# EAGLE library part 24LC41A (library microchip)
Serial EEPROM 128/512 byte, dual port
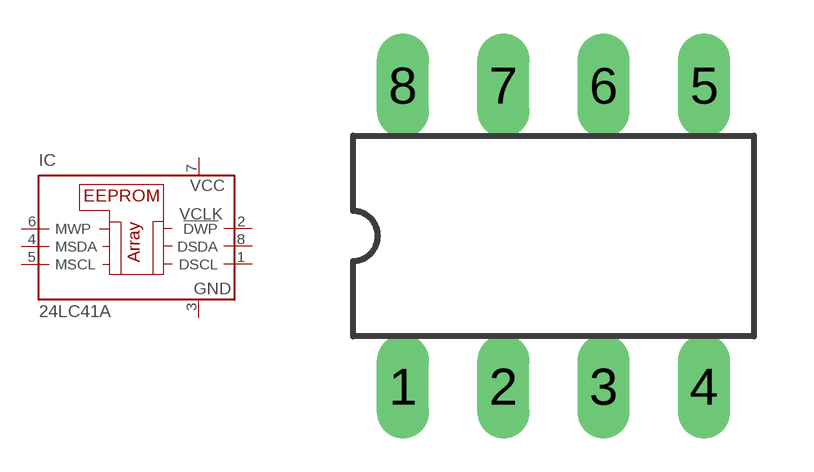
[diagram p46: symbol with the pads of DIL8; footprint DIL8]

Designator prefix IC

## 24LC41AP (OC_FARNELL: unknown; OC_NEWARK: unknown)  [DIL8]
1  DSCL  in
2  !DWP  in
3  GND  pwr
4  MSDA
5  MSCL  in
6  MWP  in
7  VCC  pwr
8  DSDA

## Footprint DIL8 (pad centres in mm)
Dual In Line package type P
drill 0.813 long: 1 -3.81,-3.81; 2 -1.27,-3.81; 3 1.27,-3.81; 4 3.81,-3.81; 5 3.81,3.81; 6 1.27,3.81; 7 -1.27,3.81; 8 -3.81,3.81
